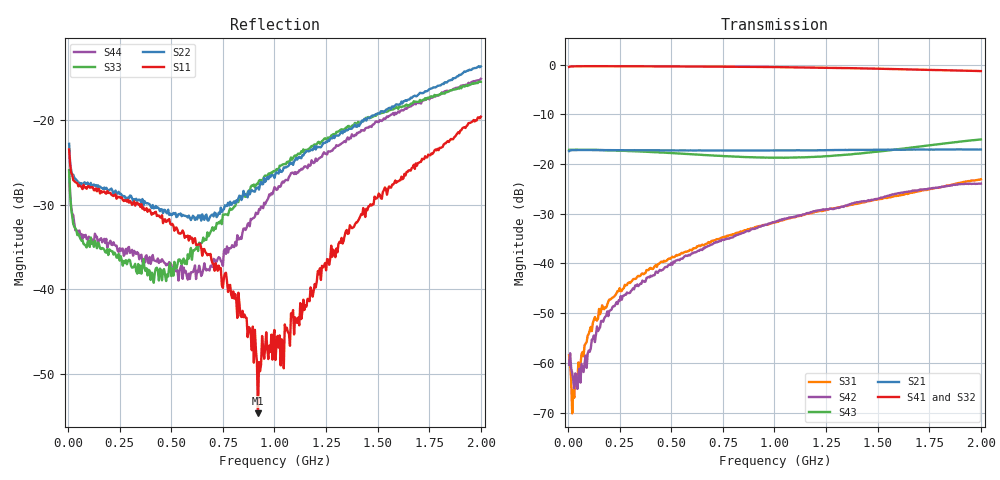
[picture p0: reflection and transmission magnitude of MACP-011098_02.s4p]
!Agilent Technologies,E5071C,MY46110647,A.11.31
!Date: Thu Jul 21 11:49:37 2022
!Data & Calibration Information:
!MACP-011098 solderedd onto PT-0003645 with F connectors, Port1 (pin3) Port2 (pin1) Port3 (pin6) Port4 (pin4)
!Freq	S11:SOLT4(ON)	S12:SOLT4(ON)	S13:SOLT4(ON)	S14:SOLT4(ON)
!	S21:SOLT4(ON)	S22:SOLT4(ON)	S23:SOLT4(ON)	S24:SOLT4(ON)
!	S31:SOLT4(ON)	S32:SOLT4(ON)	S33:SOLT4(ON)	S34:SOLT4(ON)
!	S41:SOLT4(ON)	S42:SOLT4(ON)	S43:SOLT4(ON)	S44:SOLT4(ON)
!PortZ  Port1:75+j0  Port2:75+j0  Port3:75+j0  Port4:75+j0
!Above PortZ is port z conversion or system Z0 setting when saving the data.
!When reading, reference impedance value at option line is always used.
# Hz S MA R 75
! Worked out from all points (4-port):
!   400 points, 5 MHz to 2 GHz, reference 75 ohm
!   strongest paths, dB at 5 MHz, 505 MHz, 1.005 GHz, 1.505 GHz, 2 GHz:
!     S41: -0.5, -0.4, -0.5, -0.8, -1.3
!     S32: -0.5, -0.4, -0.5, -1.0, -1.7
!     S21: -17.4, -17.3, -17.3, -17.1, -17.1
!     S43: -17.1, -17.8, -18.7, -17.5, -15.1
!     S42: -60.4, -40.3, -31.6, -26.9, -23.9
!     S31: -58.5, -38.7, -31.7, -27.1, -23.1
!   lowest |S11| = -54.7 dB at 920 MHz (marker M1), VSWR 1.00, Z = 74.7 + j0.107 ohm
!   |S11| at or under -10 dB: start of sweep to end of sweep
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5000000  0.06688 146.0  0.1354 -177.7  0.001296 -72.4  0.9464 2.1
         0.1347 -177.9  0.07222 146.9  0.9475 2.0  0.001726 -97.8
         0.001191 -99.5  0.949 1.8  0.0505 130.9  0.1375 1.2
         0.9477 1.8  0.0009537 -128.1  0.1388 2.0  0.0496 134.2
2e7  0.04756 161.2  0.138 179.4  0.0007796 -163.9  0.9577 0.3
     0.1377 179.4  0.04642 161.3  0.9574 0.3  0.0008448 -140.2
     0.0003104 -37.8  0.9595 0.2  0.02676 147.6  0.1388 0.3
     0.9588 0.2  0.0007936 -11.0  0.139 0.2  0.02804 146.3
1.5e8  0.03911 162.7  0.1384 168.4  0.003813 97.5  0.9624 -4.3
       0.1381 168.3  0.03986 175.5  0.9634 -4.2  0.00248 112.3
       0.003484 86.3  0.9654 -4.2  0.01842 178.4  0.138 -2.1
       0.9633 -4.3  0.002186 86.9  0.1381 -2.1  0.01958 151.3
4.15e8  0.02793 149.0  0.1374 148.0  0.009937 84.8  0.9593 -12.1
        0.1372 147.9  0.03005 -170.2  0.9611 -12.2  0.007563 97.2
        0.009009 82.2  0.9616 -12.2  0.01091 -144.8  0.1316 -4.7
        0.9596 -12.1  0.007581 91.6  0.1315 -4.8  0.01484 105.5
8.25e8  0.00953 122.1  0.1368 117.7  0.02104 69.8  0.9494 -24.2
        0.1367 117.6  0.03442 -116.7  0.9506 -24.5  0.01826 83.1
        0.02036 72.8  0.9478 -24.5  0.03268 -86.8  0.1183 -3.0
        0.9501 -24.2  0.01946 83.4  0.1184 -3.1  0.01971 -5.9
9.2e8  0.001848 157.1  0.1369 110.8  0.02422 65.7  0.9469 -27.1
       0.1371 110.7  0.03985 -114.2  0.9471 -27.4  0.02145 77.8
       0.02357 69.3  0.9426 -27.4  0.04173 -86.4  0.1164 -1.3
       0.947 -27.1  0.02304 79.4  0.1165 -1.2  0.02789 -27.4
2e9  0.1046 -129.8  0.139 25.3  0.07158 17.6  0.8586 -60.0
     0.1398 25.1  0.2071 -128.5  0.8271 -62.0  0.06247 13.1
     0.07009 18.7  0.8184 -61.3  0.1679 -121.2  0.1762 5.9
     0.8597 -60.0  0.06357 13.5  0.1763 5.8  0.175 -107.4
